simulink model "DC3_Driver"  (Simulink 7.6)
settings: Solver=FixedStepDiscrete  StartTime=0.0  StopTime=7  RelTol=1e-3
InitFcn:
  | clear all
  | close all
  | clc
  | Ts=2e-6;
  | delete *.mat
libraries: powerlib x4, powerlib_extras x2, electricdrivelib x1

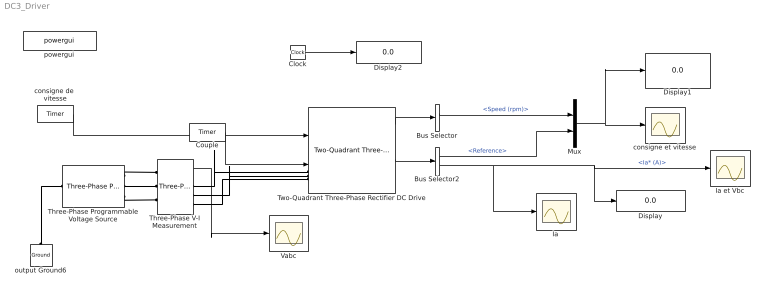
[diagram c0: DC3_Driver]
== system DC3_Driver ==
  Bus Selector : BusSelector  OutputSignals=Speed (rpm),Armature current ia (A)
  Bus Selector2 : BusSelector  OutputSignals=Reference,Ia* (A)
  Clock : Clock
  Couple : powerlib_extras/Control  Blocks/Timer  DialogController=POWERSYS.PowerSysDialog  SystemSampleTime=-1  t=[0 1.5]  e=[0 20]
  Display : Display
  Display1 : Display
  Display2 : Display
  "Ia " : Scope
  Ia et Vbc : Scope
  Mux : Mux  Inputs=2
  Three-Phase Programmable Voltage Source : powerlib/Electrical Sources/Three-Phase Programmable Voltage Source  DialogController=POWERSYS.PowerSysDialog  SystemSampleTime=-1  PositiveSequence="[380  0 60]"  VariationEntity=Amplitude  VariationType=Step  VariationStep=1  VariationRate=10  VariationMagnitude=0.3  VariationFrequency=2  VariationTiming=[6 7]  VariationPhaseA=off  Amplitudes=[1 0.8 1.2 1.0]  TimeValues=[0 0.1 0.15 0.2]  HarmonicGeneration=off  HarmonicA=[3 0.2 -25 0]  HarmonicB=[2 0.15 35 2]  Timing="[0.05  3]"
  Three-Phase V-I Measurement : powerlib/Measurements/Three-Phase V-I Measurement  DialogController=POWERSYS.PowerSysDialog  SystemSampleTime=-1  VoltageMeasurement=phase-to-ground  SetLabelV=off  LabelV=Vabc  Vpu=off  VpuLL=off  CurrentMeasurement=yes  SetLabelI=off  LabelI=Iabc  Ipu=off  Pbase=100e6  Vbase=500e3  OutputType=Complex  PhasorSimulation=off  PSBequivalent=0
  Two-Quadrant Three-Phase Rectifier DC Drive : electricdrivelib/DC drives/Two-Quadrant Three-Phase Rectifier DC Drive  SystemSampleTime=-1  showMaskWarnings=on  AverageValue=off  MechanicalLoad=Torque Tm  driveType=DC3
  Vabc : Scope
  consigne de  vitesse : powerlib_extras/Control  Blocks/Timer  DialogController=POWERSYS.PowerSysDialog  SystemSampleTime=-1  t=[0 0.2 4 5]  e=[0 200 300 0]
  consigne et vitesse : Scope
  output Ground6 : powerlib/Elements/Ground  DialogController=POWERSYS.PowerSysDialog  PhysicalDomain=powersysdomain  SubClassName=unknown  LeftPortType=p1  RightPortType=p1  LConnTagsString=a
  powergui : powerlib/powergui  Priority=2  SystemSampleTime=-1  SimulationMode=Discrete  SampleTime=Ts  frequency=60  SPID=off  DisableSnubberDevices=off  DisableRonSwitches=off  DisableVfSwitches=off  SwTol=0  Interpol=off  frequencyindice=0  echomessages=off  HookPort=off  DisplayEquations=off  FunctionMessages=off  EnableUseOfTLC=off  x0status=blocks  RestoreLinks=warning  ResistiveCurrentMeasurement=off  Frange=[0:2:500]  Ylog=off  Xlog=on  ShowGrid=off  save=off  variable=ZData  ZoomFFT=on  StartTime=0.0  cycles=1  DisplayStyle=1  fundamental=60  FreqAxis=off  MaxFrequency=1000  frequencyindicesteady=1  RmsSteady=1  display=off  Ts=0  methode=off
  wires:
  consigne de  vitesse/1 -> Two-Quadrant Three-Phase Rectifier DC Drive/1
  Two-Quadrant Three-Phase Rectifier DC Drive/1 -> Bus Selector/1
  Two-Quadrant Three-Phase Rectifier DC Drive/3 -> Bus Selector2/1
  Clock/1 -> Display2/1
  Couple/1 -> Two-Quadrant Three-Phase Rectifier DC Drive/2
  Bus Selector2/1 -> Mux/2  "<Reference>"
  Bus Selector/1 -> Mux/1  "<Speed (rpm)>"
  Mux/1 -> consigne et vitesse/1, Display1/1
  Bus Selector2/2 -> "Ia "/1, Ia et Vbc/1, Display/1  "<Ia* (A)>"
  Three-Phase V-I Measurement/1 -> Vabc/1
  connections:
  output Ground6/LConn1 -- Three-Phase Programmable Voltage Source/LConn1
  Three-Phase V-I Measurement/RConn2 -- Two-Quadrant Three-Phase Rectifier DC Drive/LConn2
  Three-Phase V-I Measurement/RConn3 -- Two-Quadrant Three-Phase Rectifier DC Drive/LConn3
  Three-Phase Programmable Voltage Source/RConn1 -- Three-Phase V-I Measurement/LConn1
  Three-Phase Programmable Voltage Source/RConn2 -- Three-Phase V-I Measurement/LConn2
  Three-Phase Programmable Voltage Source/RConn3 -- Three-Phase V-I Measurement/LConn3
  Three-Phase V-I Measurement/RConn1 -- Two-Quadrant Three-Phase Rectifier DC Drive/LConn1
